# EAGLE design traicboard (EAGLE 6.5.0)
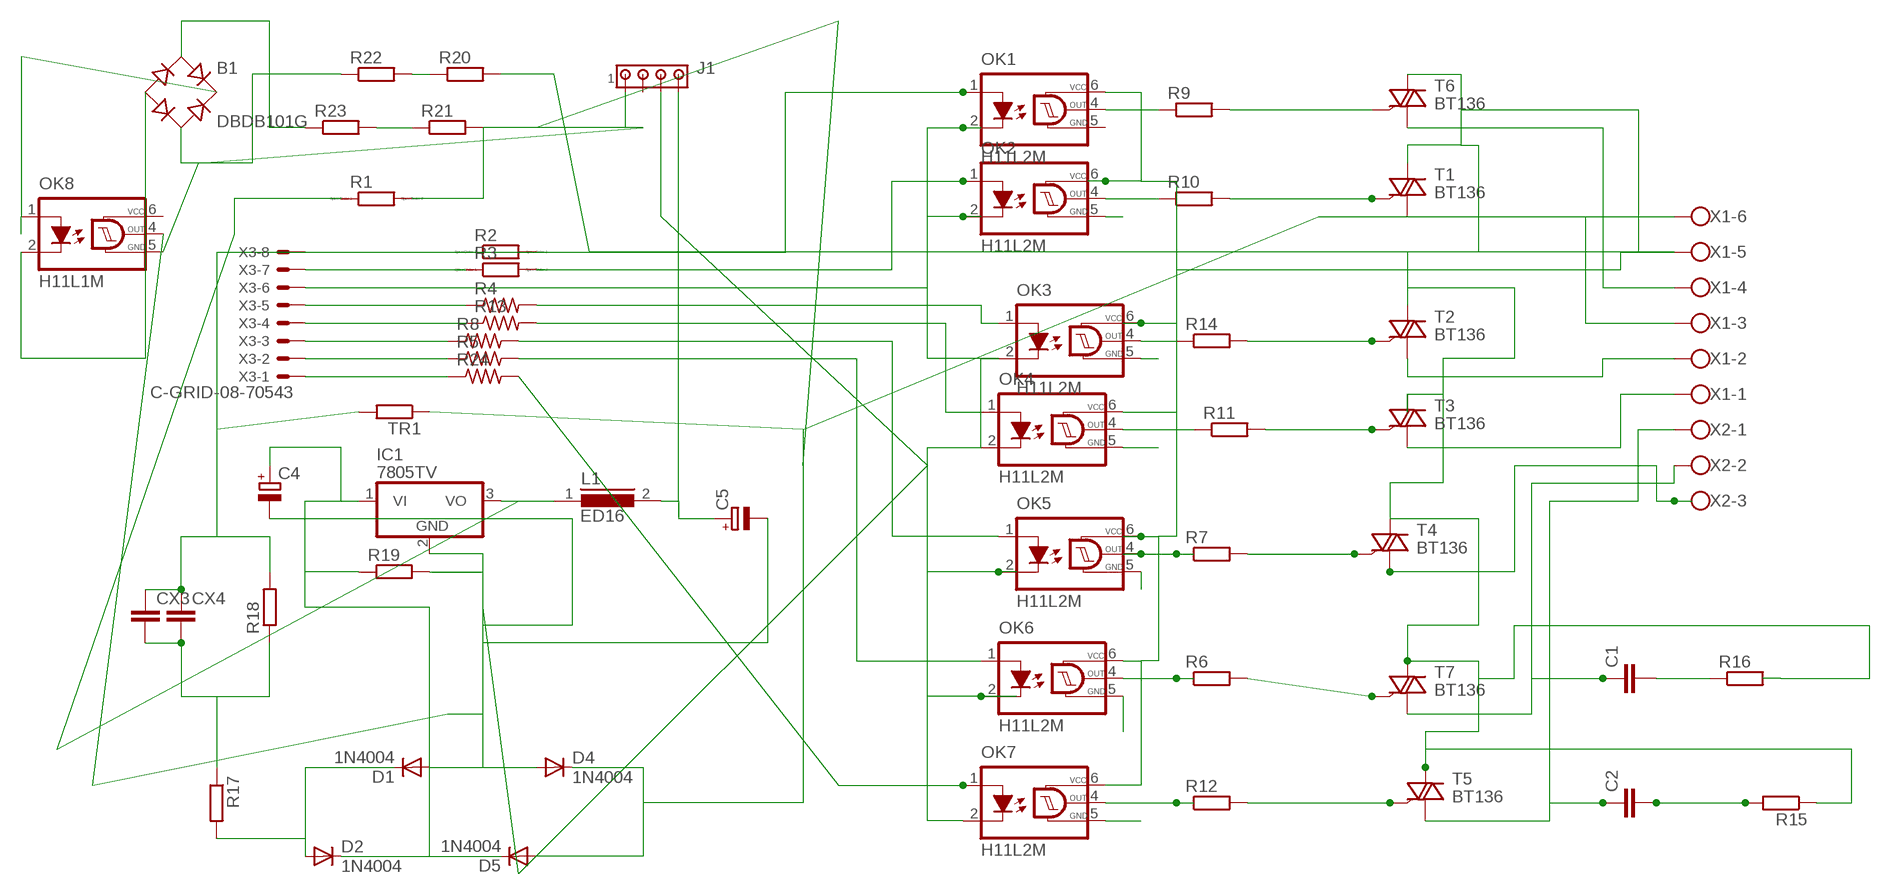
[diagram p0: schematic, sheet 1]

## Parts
B1  DBDB101G  [DB]
C1  C10/4  [C10B4]
C2  C10/4  [C10B4]
C4  CPOL-EUE2-5  [E2-5]
C5  CPOL-EUE2-5  [E2-5]
CX3  CXXC15B5  [XC15B5]
CX4  CXXC15B5  [XC15B5]
D1  1N4004  [DO41-10]
D2  1N4004  [DO41-10]
D4  1N4004  [DO41-10]
D5  1N4004  [DO41-10]
IC1  7805TV  [TO220V]
J1  MTA04-100  [10X04MTA]
L1  ED16  [ED16]
OK1  H11L2M  [DIL06]
OK2  H11L2M  [DIL06]
OK3  H11L2M  [DIL06]
OK4  H11L2M  [DIL06]
OK5  H11L2M  [DIL06]
OK6  H11L2M  [DIL06]
OK7  H11L2M  [DIL06]
OK8  H11L1M  [DIL06]
R1  R0204/7  [0204/7]
R2  R0204/7  [0204/7]
R3  R0204/7  [0204/7]
R4  R-US_0204/2V  [0204V]
R5  R-US_0204/2V  [0204V]
R6  R-EU_0204/2V  [0204V]
R7  R-EU_0204/2V  [0204V]
R8  R-US_0204/2V  [0204V]
R9  R-EU_0204/2V  [0204V]
R10  R-EU_0204/2V  [0204V]
R11  R-EU_0204/2V  [0204V]
R12  R-EU_0204/2V  [0204V]
R13  R-US_0204/2V  [0204V]
R14  R-EU_0204/2V  [0204V]
R15  R-EU_0207/5V  [0207/5V]
R16  R-EU_0207/12  [0207/12]
R17  R-EU_0207/5V  [0207/5V]
R18  R-EU_0207/10  [0207/10]
R19  R-EU_0207/5V  [0207/5V]
R20  R-EU_0309/V  [0309V]
R21  R-EU_0309/V  [0309V]
R22  R-EU_0309/V  [0309V]
R23  R-EU_0309/V  [0309V]
R24  R-US_0204/2V  [0204V]
T1  BT136  [TO220AB]
T2  BT136  [TO220AB]
T3  BT136  [TO220AB]
T4  BT136  [TO220AB]
T5  BT136  [TO220AB]
T6  BT136  [TO220AB]
T7  BT136  [TO220AB]
TR1  R-EU_0204/7  [0204/7]
X1  W237-136  [W237-136]
X2  W237-103  [W237-103]
X3  C-GRID-08-70543  [70543-08]

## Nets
N$1: OK1.1(A) R2.2
N$2: OK2.1(A) R3.2
N$3: OK3.1(A) R4.2
N$4: OK4.1(A) R13.2
N$5: OK5.1(A) R8.2
N$6: OK6.1(A) R5.2
N$7: OK7.1(A) R24.2
N$8: R2.1 X3.8
N$9: R3.1 X3.7
N$10: R4.1 X3.5
N$11: R13.1 X3.4
N$12: R8.1 X3.3
N$13: R5.1 X3.2
N$14: R24.1 X3.1
N$15: OK1.2(C) OK2.2(C) OK3.2(C) OK4.2(C) OK5.2(C) OK6.2(C) OK7.2(C) X3.6
N$16: OK1.4(OUT) R9.1
N$17: OK2.4(OUT) R10.1
N$18: OK3.4(OUT) R14.1
N$19: OK4.4(OUT) R11.1
N$20: OK5.4(OUT) R7.1
N$21: OK6.4(OUT) R6.1
N$22: OK7.4(OUT) R12.1
N$23: R9.2 T6.3(G)
N$24: R14.2 T2.3(G)
N$25: R11.2 T3.3(G)
N$26: R7.2 T4.3(G)
N$27: R6.2 T7.3(G)
N$28: R12.2 T5.3(G)
N$29: R10.2 T1.3(G)
N$30: T6.1(A1) X1.4
N$31: T4.1(A1) X2.3
N$32: T1.1(A1) X1.3
N$33: OK2.5(GND)
N$34: OK3.5(GND)
N$35: OK4.5(GND)
N$36: C1.1 T7.1(A1) X2.2
N$37: C1.2 R16.1
N$38: C2.2 R15.2
N$39: C2.1 T5.1(A1) X2.1
N$40: CX3.1 CX4.1 OK1.6(VCC) OK2.6(VCC) OK3.6(VCC) OK4.6(VCC) OK5.6(VCC) OK6.6(VCC) OK7.6(VCC) R15.1 R16.2 R18.2 R20.2 T1.2(A2) T2.2(A2) T3.2(A2) T4.2(A2) T5.2(A2) T6.2(A2) T7.2(A2) TR1.2 X1.5
N$41: T3.1(A1) X1.1
N$42: T2.1(A1) X1.2
N$43: OK5.5(GND)
N$44: OK6.5(GND)
N$45: OK7.5(GND)
N$47: CX3.2 CX4.2 R17.1 R18.1
N$48: D4.C D5.A R21.2 TR1.1 X1.6
N$49: D1.C D2.A R17.2
N$50: C5.+ J1.4 L1.2
N$51: C4.- C5.- D1.A D4.A IC1.2(GND) J1.3 OK8.4(OUT) R19.2
N$52: C4.+ D2.C D5.C IC1.1(VI) R19.1
N$55: R21.1 R23.2
N$56: R20.1 R22.2
N$58: B1.AC2 R22.1
N$59: B1.AC1 R23.1
N$60: B1.+ OK8.1(A)
N$61: B1.- OK8.2(C)
N$62: IC1.3(VO) L1.1 R1.1
N$63: J1.1 OK8.5(GND) R1.2
Unconnected: J1.2

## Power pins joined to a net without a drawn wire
GND: OK1.5(GND)
VCC: OK8.6(VCC)

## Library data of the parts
B1 = rectifier:DB?*G: Single Phase 1.0 AMP Glass Passivated Bridge Rectifier Taiwan Semiconductor Co.,Ltd. - TSC Source: http://www.taiwansemi.com/TSCbig5/ezcatfiles/cust/img/img/db101g.pdf http://www.ts.com.tw/db/pictures/modules/PDT/PDT060207001/DBLS201G.pdf
C1 C2 = capacitor-wima:C: CAPACITOR
C4 C5 = rcl:CPOL-EU: POLARIZED CAPACITOR, European symbol
CX3 CX4 = rcl:CX: X CAPACITOR
D1 D2 D4 D5 = diode:1N4004: DIODE
IC1 = linear:78*: Positive VOLTAGE REGULATOR Source: http://cache.national.com/ds/LM/LM78L05.pdf http://www.fairchildsemi.com/ds/LM/LM7805.pdf
J1 = con-amp:MTA04-100: AMP connector
L1 = inductors:ED16: INDUCTOR
OK1-OK7 = optocoupler:H11L*M: 6-Pin DIP Optocoupler Source: http://www.fairchildsemi.com/ds/H1/H11L2-M.pdf; MF: FAIRCHILD SEMICONDUCTOR; MPN: H11L2M; OC_FARNELL: 1021231; OC_NEWARK: 72K8645
OK8 = optocoupler:H11L*M: 6-Pin DIP Optocoupler Source: http://www.fairchildsemi.com/ds/H1/H11L2-M.pdf; MF: FAIRCHILD SEMICONDUCTOR; MPN: H11L1-M; OC_FARNELL: 1021127; OC_NEWARK: 72K8643
R1-R3 = eagle-ltspice:R: RESISTOR, European symbol; SPICEMODEL: NONE; SPICEPREFIX: R
R4 R5 R8 R13 R24 = rcl:R-US_: RESISTOR, American symbol
R6 R7 R9-R12 R14-R23 TR1 = rcl:R-EU_: RESISTOR, European symbol
T1-T7 = triac:BT136: Triac BT136 series E sensitive gate Source: http://www.nxp.com/acrobat_download/datasheets/BT136_SERIES_E_2.pdf
X1 = con-wago-500:W237-136: WAGO SCREW CLAMP; MPN: 237-136; OC_FARNELL: unknown; OC_NEWARK: 84K9151
X2 = con-wago-500:W237-103: WAGO SCREW CLAMP; MPN: 237-103; OC_FARNELL: unknown; OC_NEWARK: 18M7116
X3 = con-molex:C-GRID-08: CONNECTOR wire to board 2.54 mm (0.100") pitch header; OC_FARNELL: unknown; OC_NEWARK: unknown

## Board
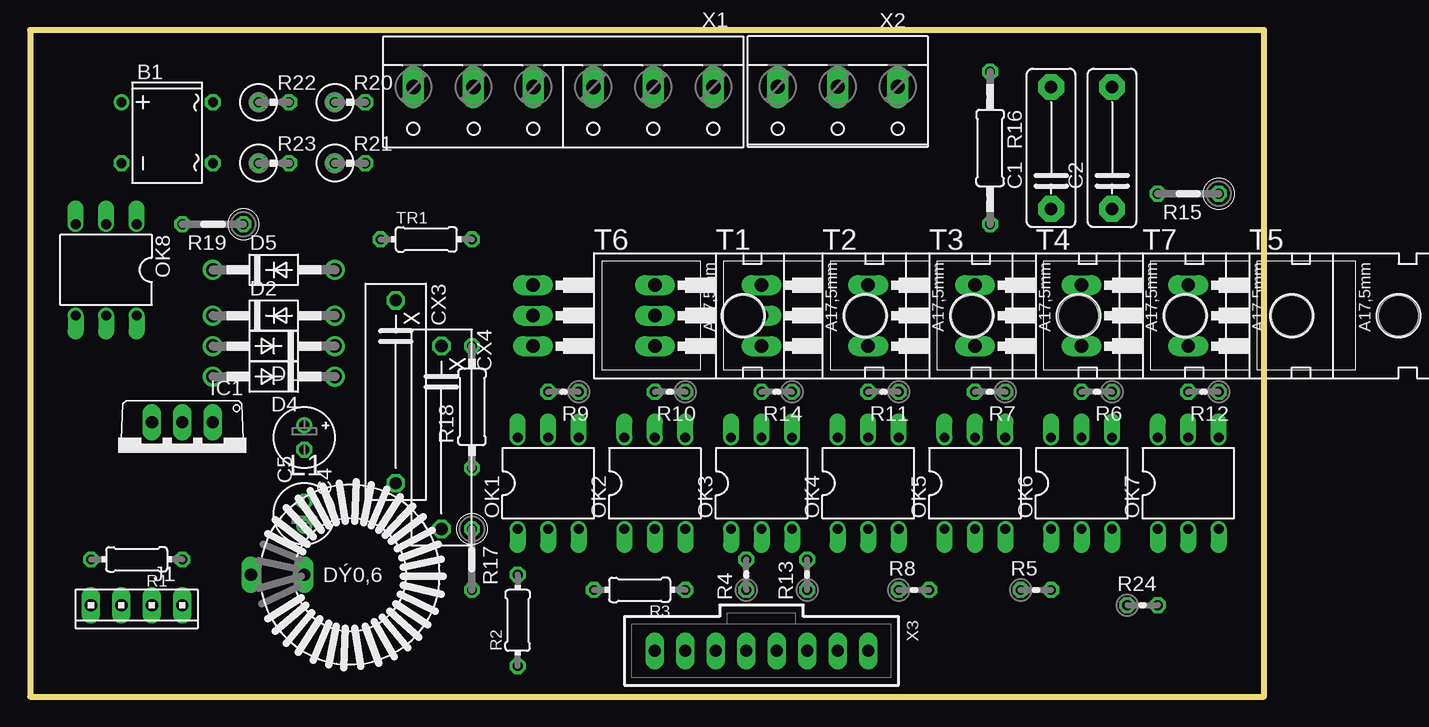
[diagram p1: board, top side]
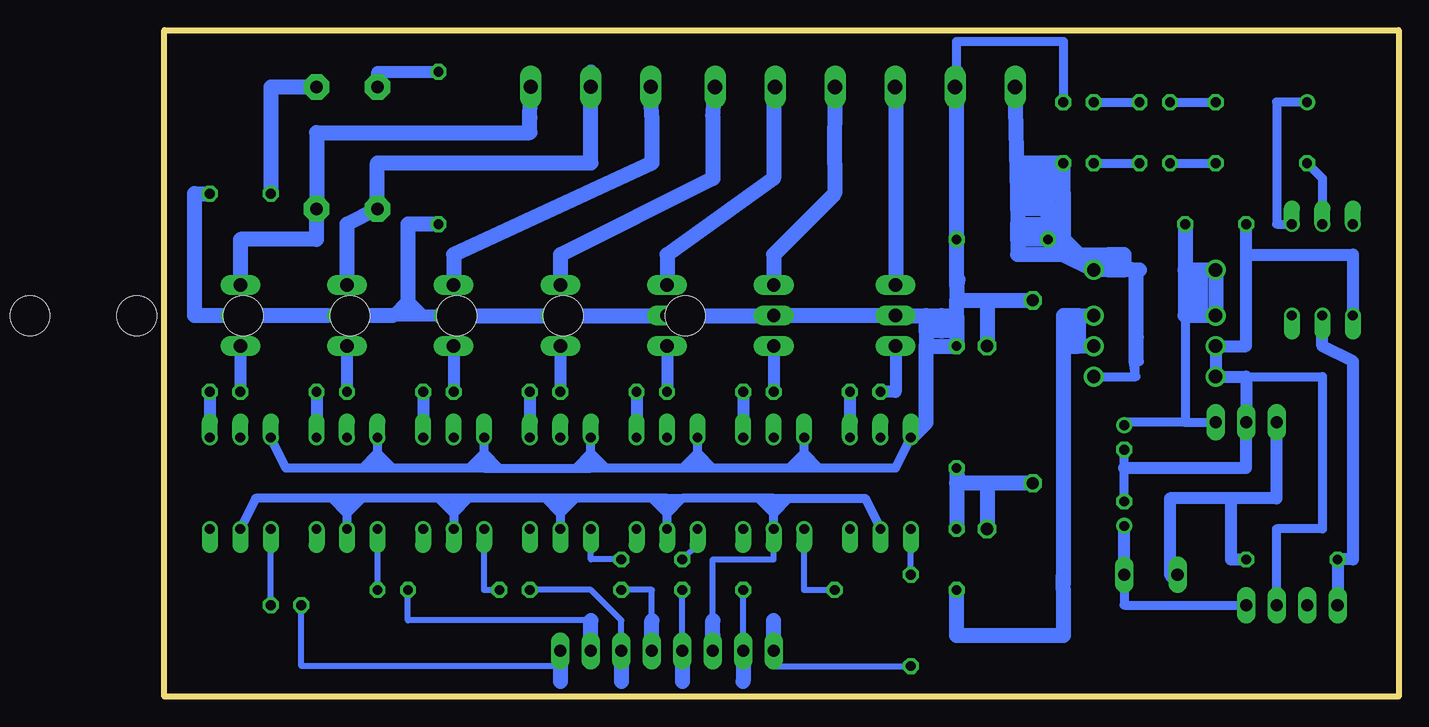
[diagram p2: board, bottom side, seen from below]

Size 102.85 x 55.55 mm. Coordinates in mm from the lower left corner, seen from the top.
Outline: 0,0 102.85,0 102.85,55.55 0,55.55 0,0
Copper layers (1*16): Top 0.035mm / dielectric 1.5mm / Bottom 0.035mm
Design rules "default": minimum track width 10mil, minimum drill 24mil, track to track 8mil, track to pad 8mil, pad to pad 8mil, via to via 8mil, smd to smd 8mil, copper to edge 40mil, drill to drill 8mil, minimum pad ring 10mil, minimum via ring 8mil, stop-mask expansion 4mil, vias tented up to drill 0mil, thermal gap 10mil

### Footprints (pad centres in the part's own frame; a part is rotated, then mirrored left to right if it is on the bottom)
DB = drill 0.813: + -2.54,-3.81 | drill 0.813 octagon: - 2.54,-3.81; AC1 2.54,3.81; AC2 -2.54,3.81
C10B4 = drill 1.016 pad 2.159 octagon: 1 -5.08,0; 2 5.08,0
E2-5 = drill 0.813 pad 1.27: + -1.016,0 | drill 0.813 pad 1.27 octagon: - 1.016,0
XC15B5 = drill 1.016 octagon: 1 -7.62,0; 2 7.62,0
DO41-10 = drill 1.118: A 5.08,0; C -5.08,0
TO220V = drill 1.016 long: 1 -2.54,-2.54; 2 0,-2.54; 3 2.54,-2.54
10X04MTA = drill 1.016 long: 1 3.81,0; 2 1.27,0; 3 -1.27,0; 4 -3.81,0
ED16 = drill 1.016 long: 1 -8.255,0; 2 -3.81,0
DIL06 = drill 0.813 offset: 1 -2.54,-3.81; 2 0,-3.81; 3 2.54,-3.81; 4 2.54,3.81; 5 0,3.81; 6 -2.54,3.81
0204/7 = drill 0.813 octagon: 1 -3.81,0; 2 3.81,0
0204V = drill 0.813 octagon: 1 -1.27,0; 2 1.27,0
0207/5V = drill 0.813 octagon: 1 -2.54,0; 2 2.54,0
0207/12 = drill 0.813 octagon: 1 -6.35,0; 2 6.35,0
0207/10 = drill 0.813 octagon: 1 -5.08,0; 2 5.08,0
0309V = drill 0.813 octagon: 1 -1.27,0; 2 1.27,0
TO220AB = drill 1.118 long: 1 -2.54,-6.35; 2 0,-6.35; 3 2.54,-6.35 | hole 3.302: 0,11.176
W237-136 = drill 1.194 long: 1 -12.5,-1.27; 2 -7.5,-1.27; 3 -2.5,-1.27; 4 2.5,-1.27; 5 7.5,-1.27; 6 12.5,-1.27
W237-103 = drill 1.194 long: 1 -5,-1.29; 2 0,-1.29; 3 5,-1.29
70543-08 = drill 1.016 long: 1 -8.89,0; 2 -6.35,0; 3 -3.81,0; 4 -1.27,0; 5 1.27,0; 6 3.81,0; 7 6.35,0; 8 8.89,0

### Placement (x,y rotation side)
B1  11.43,46.99 270 top
C1  85.09,45.72 90 top
C2  90.17,45.72 90 top
C4  22.86,21.59 270 top
C5  22.86,15.24 90 top
CX3  30.48,25.4 270 top
CX4  34.29,21.59 270 top
D1  20.32,29.21 180 top
D2  20.32,31.75 0 top
D4  20.32,26.67 180 top
D5  20.32,35.56 0 top
IC1  12.7,20.32 180 top
J1  8.89,7.62 180 top
L1  26.67,10.16 0 top
OK1  43.18,17.78 0 top
OK2  52.07,17.78 0 top
OK3  60.96,17.78 0 top
OK4  69.85,17.78 0 top
OK5  78.74,17.78 0 top
OK6  87.63,17.78 0 top
OK7  96.52,17.78 0 top
OK8  6.35,35.56 180 top
R1  8.89,11.43 180 top
R2  40.64,6.35 90 top
R3  50.8,8.89 180 top
R4  59.69,10.16 90 top
R5  83.82,8.89 0 top
R6  88.9,25.4 180 top
R7  80.01,25.4 180 top
R8  73.66,8.89 0 top
R9  44.45,25.4 180 top
R10  53.34,25.4 180 top
R11  71.12,25.4 180 top
R12  97.79,25.4 180 top
R13  64.77,10.16 90 top
R14  62.23,25.4 180 top
R15  96.52,41.91 180 top
R16  80.01,45.72 270 top
R17  36.83,11.43 270 top
R18  36.83,24.13 90 top
R19  15.24,39.37 180 top
R20  26.67,49.53 0 top
R21  26.67,44.45 0 top
R22  20.32,49.53 0 top
R23  20.32,44.45 0 top
R24  92.71,7.62 0 top
T1  58.42,31.75 270 top
T2  67.31,31.75 270 top
T3  76.2,31.75 270 top
T4  85.09,31.75 270 top
T5  102.87,31.75 270 top
T6  48.26,31.75 270 top
T7  93.98,31.75 270 top
TR1  33.02,38.1 0 top
X1  44.45,49.53 180 top
X2  67.31,49.53 180 top
X3  60.96,3.81 180 top

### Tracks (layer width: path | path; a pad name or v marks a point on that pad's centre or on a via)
N$1
  Bottom 0.508: R2.2 OK1.1
N$2
  Bottom 0.508: OK2.1 49.53,8.89 R3.2
N$3
  Bottom 0.508: OK3.1 58.42,12.7 R4.2
N$4
  Bottom 0.508: R13.2 67.31,11.43 OK4.1
N$5
  Bottom 0.508: OK5.1 76.2,8.89 R8.2
N$6
  Bottom 0.508: OK6.1 R5.2
N$7
  Bottom 0.508: R24.2 OK7.1
N$8
  Bottom 0.508: X3.8 52.07,2.54 R2.1
  Bottom 1.27: X3.8 52.07,6.35
N$9
  Bottom 0.508: X3.7 R3.1
  Bottom 1.27: X3.7 54.61,1.27
N$10
  Bottom 0.508: X3.5 R4.1
  Bottom 1.27: X3.5 59.69,1.27
N$11
  Bottom 0.508: R13.1 62.23,8.89 62.23,6.35
  Bottom 1.27: X3.4 62.23,6.35
N$12
  Bottom 0.508: R8.1 67.31,8.89 64.77,6.35 X3.3
  Bottom 1.27: X3.3 64.77,1.27
N$13
  Bottom 0.508: R5.1 82.55,6.35 67.31,6.35
  Bottom 1.27: X3.2 67.31,6.35
N$14
  Bottom 0.508: R24.1 91.44,2.54 69.85,2.54
  Bottom 1.27: X3.1 69.85,2.54 69.85,1.27
N$15
  Bottom 0.025: OK3.2 60.96,13.34
  Bottom 0.406: 57.15,5.08 57.15,6.35 | OK2.2 52.07,16.51
  Bottom 0.508: 57.15,6.35 57.15,11.43 52.07,11.43 OK2.2
  Bottom 0.762: OK1.2 44.45,16.51 50.8,16.51 | 52.07,16.51 50.8,16.51 | OK2.2 52.07,15.24 | 52.07,15.24 52.07,16.51 | 60.96,16.51 60.96,15.24 | 52.07,16.51 59.69,16.51 | 69.85,16.51 69.85,15.24 | 69.85,15.24 OK4.2 | 60.96,16.51 62.23,16.51 | 62.23,16.51 68.58,16.51 | 68.58,16.51 69.85,16.51 | 78.74,16.51 78.74,15.24 | 78.74,15.24 OK5.2 | 69.85,16.51 71.12,16.51 | 71.12,16.51 77.47,16.51 | 77.47,16.51 78.74,16.51 | 87.63,16.51 87.63,15.24 | 87.63,15.24 OK6.2 | 78.74,16.51 80.01,16.51 | 80.01,16.51 86.36,16.51 | 86.36,16.51 87.63,16.51 | OK7.2 95.25,16.51 88.9,16.51 | 87.63,16.51 88.9,16.51 | 50.8,16.51 52.07,15.24 | 52.07,15.24 53.34,16.51 | 59.69,16.51 60.96,15.24 | 60.96,15.24 62.23,16.51 | 68.58,16.51 69.85,15.24 | 69.85,15.24 71.12,16.51 | 77.47,16.51 78.74,15.24 | 78.74,15.24 80.01,16.51 | 86.36,16.51 87.63,15.24 | 87.63,15.24 88.9,16.51 | OK3.2 60.96,15.24 | 60.96,16.51 59.69,16.51
  Bottom 1.27: 57.15,5.08 X3.6 57.15,6.35
N$16
  Bottom 1.016: R9.1 OK1.4
N$17
  Bottom 1.016: R10.1 OK2.4
N$18
  Bottom 1.016: R14.1 OK3.4
N$19
  Bottom 1.016: R11.1 OK4.4
N$20
  Bottom 1.016: R7.1 OK5.4
N$21
  Bottom 1.016: R6.1 OK6.4
N$22
  Bottom 1.016: R12.1 OK7.4
N$23
  Bottom 1.016: T6.3 41.91,25.4 R9.2
N$24
  Bottom 1.016: T2.3 R14.2
N$25
  Bottom 1.016: T3.3 R11.2
N$26
  Bottom 1.016: T4.3 R7.2
N$27
  Bottom 1.016: T7.3 R6.2
N$28
  Bottom 1.016: T5.3 R12.2
N$29
  Bottom 1.016: T1.3 R10.2
N$30
  Bottom 1.016: 41.91,50.8 X1.4
  Bottom 1.27: 41.91,50.8 T6.1
N$31
  Bottom 1.27: T4.1 78.74,36.83 62.23,44.45 62.23,48.26 X2.3
N$32
  Bottom 1.27: T1.1 52.07,36.83 46.99,41.91 46.99,44.45 X1.3
N$36
  Bottom 0.254: 67.31,52.07 X2.2
  Bottom 1.27: 67.31,52.07 67.31,44.45 85.09,44.45 C1.1 87.63,39.37 T7.1
N$37
  Bottom 1.016: C1.2 85.09,52.07 R16.1
N$38
  Bottom 1.27: C2.2 93.98,50.8 R15.2
N$39
  Bottom 1.27: X2.1 72.39,48.26 72.39,46.99 90.17,46.99 C2.1 90.17,38.1 96.52,38.1 T5.1
N$40
  Bottom 0.254: T6.2 T7.2 | 36.83,52.07 X1.5 | 33.02,33.02 34.29,33.02 36.83,33.02 36.83,34.78 36.73,34.78
  Bottom 0.762: 48.26,19.05 41.91,19.05 OK1.6 | 48.26,19.05 49.53,19.05 | 49.53,19.05 49.53,20.32 | 49.53,20.32 OK2.6 | 49.53,19.05 50.8,19.05 | 50.8,19.05 57.15,19.05 | 57.15,19.05 58.42,19.05 | 58.42,19.05 58.42,20.32 | 58.42,20.32 OK3.6 | 67.31,19.05 67.31,20.32 | 67.31,20.32 OK4.6 | 58.42,19.05 59.69,19.05 | 59.69,19.05 66.04,19.05 | 66.04,19.05 67.31,19.05 | 76.2,19.05 76.2,20.32 | 76.2,20.32 OK5.6 | 76.2,19.05 77.47,19.05 | 77.47,19.05 83.82,19.05 | 83.82,19.05 85.09,19.05 | OK7.6 92.71,19.05 86.36,19.05 | 85.09,19.05 86.36,19.05 | OK6.6 85.09,20.32 | 85.09,20.32 85.09,19.05 | 76.2,19.05 74.93,19.05 | 74.93,19.05 68.58,19.05 | 68.58,19.05 67.31,19.05 | 48.26,19.05 49.53,20.32 | 49.53,20.32 50.8,19.05 | 57.15,19.05 58.42,20.32 | 58.42,20.32 59.69,19.05 | 66.04,19.05 67.31,20.32 | 67.31,20.32 68.58,19.05 | 74.93,19.05 76.2,20.32 | 76.2,20.32 77.47,19.05 | 83.82,19.05 85.09,20.32 | 85.09,20.32 86.36,19.05 | 36.83,52.07 36.83,54.61 27.94,54.61 R20.2
  Bottom 1.016: T4.2 81.28,31.75 | 81.28,31.75 82.55,31.75 | 82.55,31.75 83.82,31.75 82.55,33.02 | 82.55,33.02 82.55,31.75 | 81.28,31.75 82.55,33.02
  Bottom 1.27: OK1.6 39.37,22.86 39.37,29.21 | 39.37,30.48 39.37,31.75 | R15.1 100.33,41.91 100.33,31.75 T7.2 | 36.83,34.29 TR1.2 36.83,52.07 | 39.37,31.75 T6.2 T1.2 T2.2 T3.2 T4.2 | 39.37,31.75 38.1,31.75 | 83.82,31.75 T7.2 | T7.2 T5.2 | R16.2 82.55,39.37 82.55,33.02 | 36.83,31.75 36.83,30.48 | 36.83,30.48 R18.2 39.37,29.21 | 38.1,31.75 36.83,31.75 | 36.83,31.75 36.83,33.02 | 36.73,34.78 36.83,34.29 | 36.83,34.29 36.83,33.02 | 36.83,33.02 CX3.1 | 38.1,31.75 38.1,30.48 | 36.83,30.48 38.1,30.48 | 38.1,30.48 39.37,30.48 | 39.37,30.48 39.37,29.21 | 34.29,33.02 CX4.1
N$41
  Bottom 1.27: T3.1 69.85,36.83 57.15,43.18 57.15,48.26 X1.1
N$42
  Bottom 1.27: T2.1 60.96,36.83 52.07,43.18 52.07,49.53 X1.2
N$47
  Bottom 0.254: 34.29,17.78 33.02,17.78 36.73,18.27
  Bottom 1.27: R17.1 R18.1 36.73,18.27 36.83,17.78 CX3.2 | 34.29,17.78 CX4.2
N$48
  Bottom 0.003: 21.89,26.67 21.59,26.97 | 21.59,26.97 21.59,29.95 | 21.59,26.97 D4.C
  Bottom 0.762: 29.21,44.45 30.48,43.18 31.75,41.91 31.75,44.45 | 22.12,27.94 21.89,26.67 D4.C | 22.12,27.94 22.12,35.56 | 22.12,27.94 21.59,27.94 21.59,29.95 21.59,35.56 | 24.13,35.56 31.75,39.37 31.75,48.26
  Bottom 1.27: 27.94,41.91 27.94,40.64 | 27.94,40.64 29.21,39.37 | 29.21,39.37 TR1.1 | 27.94,41.91 29.21,41.91 | 29.21,41.91 31.75,41.91 | 31.75,41.91 X1.6 | 29.21,40.64 31.75,40.64 | 31.75,40.64 31.75,41.91 | 31.75,40.64 31.75,39.37 | 31.75,39.37 29.21,39.37 | 27.94,41.91 R21.2 | R21.2 29.21,44.45 | 29.21,44.45 31.75,44.45 30.48,43.18 29.21,43.18 R21.2 | D5.A 27.94,36.83 | 27.94,36.83 TR1.1 | TR1.1 D5.A | 21.59,35.56 22.12,35.56 22.86,35.56 | 24.13,35.56 D5.A | 29.21,40.64 27.94,40.64 | TR1.1 31.75,38.1 | 31.75,38.1 31.75,36.83 27.94,36.83 | 31.75,38.1 31.75,39.37 | D5.A 27.94,38.1 | 27.94,38.1 29.21,39.37 | 29.21,39.37 29.21,40.64 | 29.21,40.64 29.21,41.91 | 29.21,41.91 29.21,44.45 | 27.94,40.64 27.94,38.1 | 27.94,38.1 27.94,36.83 | 27.94,36.83 24.13,36.83 | 24.13,36.83 24.13,35.56 | 24.13,35.56 22.86,35.56 | 22.86,35.56 22.86,36.83 24.13,36.83
N$49
  Bottom 0: 27.94,9.42 28.47,13.97
  Bottom 0.003: 28.47,13.97 27.94,8.89
  Bottom 1.27: 26.67,31.75 27.94,31.75 27.94,29.21 | 27.94,29.21 27.94,9.42 | 27.94,10.16 27.94,8.89 27.94,5.08 36.83,5.08 R17.2 | D1.C 26.67,29.21 | 26.67,31.75 D2.A | 26.67,29.21 26.67,31.75 | 27.94,29.21 26.67,29.21
N$50
  Bottom 0.762: J1.4 22.86,7.62 L1.2
  Bottom 1.016: L1.2 C5.+
N$51
  Bottom 0.762: 12.7,26.67 6.35,26.67 6.35,13.97 10.16,13.97 J1.3 | C4.- 22.86,19.05 C5.-
  Bottom 1.016: 12.7,36.83 12.7,29.21 D1.A D4.A 12.7,26.67 IC1.2 12.7,19.05 22.86,19.05 | 12.7,36.83 R19.2 | OK8.4 3.81,36.83 12.7,36.83
N$52
  Bottom 0.762: 17.78,31.75 17.78,22.86 | 17.78,22.86 22.86,22.86 C4.+ | 17.78,22.86 IC1.1
  Bottom 1.27: R19.1 17.78,35.56 | 17.78,35.56 16.51,35.56 | 17.78,35.56 17.78,31.75 | 17.78,31.75 16.51,35.56 | 16.51,35.56 D5.C D2.C 16.51,31.75 | 16.51,31.75 17.78,31.75 | 16.51,35.56 16.51,31.75
N$55
  Bottom 0.762: R21.1 R23.2
N$56
  Bottom 0.762: R20.1 R22.2
N$58
  Bottom 0.762: R22.1 B1.AC2
N$59
  Bottom 0.762: R23.1 B1.AC1
N$60
  Bottom 0.762: B1.+ 10.16,49.53 10.16,39.37 OK8.1
N$61
  Bottom 0.762: OK8.2 6.35,43.18 B1.-
N$62
  Bottom 1.016: 13.97,16.51 19.05,16.51 19.05,10.16 18.41,9.52 L1.1 | IC1.3 10.16,16.51 13.97,16.51 | 13.97,16.51 13.97,11.43 R1.1
N$63
  Bottom 1.016: OK8.5 6.35,29.21 3.81,27.94 3.81,11.43 R1.2 J1.1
